// TwinCAT 3 PLC project Untitled1
// ProgramVersion: 3.1.4024.0
// CompilerDefines: VISU_USEWSTRING
// libraries:
//   CmpBitmapPool, * (System)
//   GearMotionBaseApplication, * (Beckhoff_sh Yuyang)
//   Tc2_EtherCAT, * (Beckhoff Automation GmbH)
//   Tc2_Math, * (Beckhoff Automation GmbH)
//   Tc2_MC2, * (Beckhoff Automation GmbH)
//   Tc2_MC2_Camming, * (Beckhoff Automation GmbH)
//   Tc2_Standard, * (Beckhoff Automation GmbH)
//   Tc2_System, * (Beckhoff Automation GmbH)
//   Tc2_Utilities, * (Beckhoff Automation GmbH)
//   Tc3_MC2_AdvancedHoming, * (Beckhoff Automation GmbH)
//   Tc3_Module, * (Beckhoff Automation GmbH)
//   VisuSymbols,3.5.10.0,System
// project tree:
//   / GlobalTextList.TcGTLO, PhysicalDisplay.TcIPO, VISU_TASK.TcTTO, Param.TcGVL, PlcTask.TcTTO, 视图管理器.TcVMO
//   Visus/ FB_Visus.TcPOU, Visualization.TcVIS
//   _04_Application/ MAIN.TcPOU
//   _03_MotionSystem/ FB_ShowMotion.TcPOU, I_ShowMotion.TcIO
// real-time tasks:
//   TASK PlcTask: cycle T#10ms, priority 20, ADS port 350
//   TASK VISU_TASK: cycle T#200000us, priority 30, ADS port 351
// motion (NC):
//   TASK NC-Task 1 SAF: cycle T#2ms, priority 4, ADS port 501
//   TASK NC-Task 1 SVB: cycle T#10ms, priority 8, ADS port 511
//   AXIS Axis 1_S (id 1)
//     Dynamic: Acceleration=14565, Deceleration=14565, Jerk=7282.5
//     Velo: RefSearch=291.3, RefSync=291.3, SlowManual=300, Fast=29130, Maximum=29130
//     OtherSettings: AllowMotionCmdToSlave=true
//     encoder EncType=1
//       EncPara: ScaleFactorNumerator=360, ScaleFactorDenominator=1048576, Offset=4873.63
//     drive DrvType=5
//       Analog: VeloReferenz=32043, TorqueSetpointScale=10, ScaleFactorActTorque=0.1
//       TimeComp: TaskDelayCycles=1
//     controller CtrType=1
//       CtrPara: PriorControlFactor=1
//         Observer: BandWidth=20
//   AXIS Axis 2_E (id 2)
//     Dynamic: Acceleration=14565, Deceleration=14565, Jerk=7282.5
//     Velo: RefSearch=291.3, RefSync=291.3, SlowManual=300, Fast=29130, Maximum=29130
//     OtherSettings: AllowMotionCmdToSlave=true
//     encoder EncType=1
//       EncPara: ScaleFactorNumerator=360, ScaleFactorDenominator=1048576, Offset=-6850.4
//     drive DrvType=5
//       Analog: VeloReferenz=32043, TorqueSetpointScale=10, ScaleFactorActTorque=0.1
//       TimeComp: TaskDelayCycles=1
//     controller CtrType=1
//       CtrPara: PriorControlFactor=1
//         Observer: BandWidth=20
//   AXIS Axis 3_R (id 3)
//     Dynamic: Acceleration=43695, Deceleration=43695, Jerk=131085
//     Velo: RefSearch=291.3, RefSync=291.3, SlowManual=1456.5, FastManual=8739, Fast=29130, Maximum=29130
//     OtherSettings: AllowMotionCmdToSlave=true
//     encoder EncType=1
//       EncPara: ScaleFactorNumerator=360, ScaleFactorDenominator=1048576, Offset=-4097.87
//     drive DrvType=5
//       Analog: VeloReferenz=32043, TorqueSetpointScale=10, ScaleFactorActTorque=0.1
//       TimeComp: TaskDelayCycles=1
//     controller CtrType=1
//       CtrPara: PriorControlFactor=1
//         PosDiffControl: Enable=false
//         Observer: BandWidth=20
//   AXIS Axis 4_V (id 4)
//     Dynamic: Acceleration=14565, Deceleration=14565, Jerk=7282.5
//     Velo: RefSearch=291.3, RefSync=291.3, SlowManual=300, Fast=29130, Maximum=29130
//     OtherSettings: AllowMotionCmdToSlave=true
//     encoder EncType=1
//       EncPara: ScaleFactorNumerator=360, ScaleFactorDenominator=1048576, Offset=-3588.52
//     drive DrvType=5
//       Analog: VeloReferenz=32043, TorqueSetpointScale=10, ScaleFactorActTorque=0.1
//       TimeComp: TaskDelayCycles=1
//     controller CtrType=1
//       CtrPara: PriorControlFactor=1
//         Observer: BandWidth=20
//   AXIS Axis 5_O (id 5)
//     Dynamic: Acceleration=14565, Deceleration=14565, Jerk=7282.5
//     Velo: RefSearch=291.3, RefSync=291.3, SlowManual=300, Fast=29130, Maximum=29130
//     OtherSettings: AllowMotionCmdToSlave=true
//     encoder EncType=1
//       EncPara: ScaleFactorNumerator=360, ScaleFactorDenominator=1048576, Offset=-612.17
//     drive DrvType=5
//       Analog: VeloReferenz=32043, TorqueSetpointScale=10, ScaleFactorActTorque=0.1
//       TimeComp: TaskDelayCycles=1
//     controller CtrType=1
//       CtrPara: PriorControlFactor=1
//         Observer: BandWidth=20
//   AXIS Axis 6 (id 6)
//     OtherSettings: AllowMotionCmdToSlave=true
//     encoder EncType=19
//       EncPara: MaxCount=#xffffffff
//     drive DrvType=16
//       DrvPara: MaxCount=#xffffffff, DriveControlDWord=#x00000100
//         Analog: TorqueSetpointScale=10, ScaleFactorActTorque=0.1
//         TimeComp: TaskDelayCycles=1
//     controller CtrType=1
//       CtrPara: PriorControlFactor=1
//         Observer: BandWidth=20
//   AXIS Axis 7 (id 7)
//     OtherSettings: AllowMotionCmdToSlave=true
//     encoder EncType=19
//       EncPara: MaxCount=#xffffffff
//     drive DrvType=16
//       DrvPara: MaxCount=#xffffffff, DriveControlDWord=#x00000100
//         Analog: TorqueSetpointScale=10, ScaleFactorActTorque=0.1
//         TimeComp: TaskDelayCycles=1
//     controller CtrType=1
//       CtrPara: PriorControlFactor=1
//         Observer: BandWidth=20
//   AXIS Axis 8 (id 8)
//     OtherSettings: AllowMotionCmdToSlave=true
//     encoder EncType=19
//       EncPara: MaxCount=#xffffffff
//     drive DrvType=16
//       DrvPara: MaxCount=#xffffffff, DriveControlDWord=#x00000100
//         Analog: TorqueSetpointScale=10, ScaleFactorActTorque=0.1
//         TimeComp: TaskDelayCycles=1
//     controller CtrType=1
//       CtrPara: PriorControlFactor=1
//         Observer: BandWidth=20
// variable links:
//   Untitled1/Untitled1 Instance <-> NC-Task 1 SAF/Axes/Axis 1_S
//     PlcTask Inputs/MAIN.fbShowMotion.Axisinstance[1].NcToPlc <-> Outputs/ToPlc
//     PlcTask Inputs/MAIN.fbVisus.ArrAxisNotMoving[1] <-> Outputs/ToPlc/StateDWord/NotMoving
//     PlcTask Inputs/MAIN.fbVisus.ArrAxisPosition[1] <-> Outputs/ToPlc/ActPos
//     PlcTask Outputs/MAIN.fbShowMotion.Axisinstance[1].PlcToNc <-> Inputs/FromPlc
//   Untitled1/Untitled1 Instance <-> NC-Task 1 SAF/Axes/Axis 2_E
//     PlcTask Inputs/MAIN.fbShowMotion.Axisinstance[2].NcToPlc <-> Outputs/ToPlc
//     PlcTask Inputs/MAIN.fbVisus.ArrAxisNotMoving[2] <-> Outputs/ToPlc/StateDWord/NotMoving
//     PlcTask Inputs/MAIN.fbVisus.ArrAxisPosition[2] <-> Outputs/ToPlc/ActPos
//     PlcTask Outputs/MAIN.fbShowMotion.Axisinstance[2].PlcToNc <-> Inputs/FromPlc
//   Untitled1/Untitled1 Instance <-> NC-Task 1 SAF/Axes/Axis 3_R
//     PlcTask Inputs/MAIN.fbShowMotion.Axisinstance[3].NcToPlc <-> Outputs/ToPlc
//     PlcTask Inputs/MAIN.fbVisus.ArrAxisNotMoving[3] <-> Outputs/ToPlc/StateDWord/NotMoving
//     PlcTask Inputs/MAIN.fbVisus.ArrAxisPosition[3] <-> Outputs/ToPlc/ActPos
//     PlcTask Outputs/MAIN.fbShowMotion.Axisinstance[3].PlcToNc <-> Inputs/FromPlc
//   Untitled1/Untitled1 Instance <-> NC-Task 1 SAF/Axes/Axis 4_V
//     PlcTask Inputs/MAIN.fbShowMotion.Axisinstance[4].NcToPlc <-> Outputs/ToPlc
//     PlcTask Inputs/MAIN.fbVisus.ArrAxisNotMoving[4] <-> Outputs/ToPlc/StateDWord/NotMoving
//     PlcTask Inputs/MAIN.fbVisus.ArrAxisPosition[4] <-> Outputs/ToPlc/ActPos
//     PlcTask Outputs/MAIN.fbShowMotion.Axisinstance[4].PlcToNc <-> Inputs/FromPlc
//   Untitled1/Untitled1 Instance <-> NC-Task 1 SAF/Axes/Axis 5_O
//     PlcTask Inputs/MAIN.fbShowMotion.Axisinstance[5].NcToPlc <-> Outputs/ToPlc
//     PlcTask Inputs/MAIN.fbVisus.ArrAxisNotMoving[5] <-> Outputs/ToPlc/StateDWord/NotMoving
//     PlcTask Inputs/MAIN.fbVisus.ArrAxisPosition[5] <-> Outputs/ToPlc/ActPos
//     PlcTask Outputs/MAIN.fbShowMotion.Axisinstance[5].PlcToNc <-> Inputs/FromPlc

CONFIGURATION Untitled1
    RESOURCE PLC ON TwinCAT3
        TASK VISU_TASK(INTERVAL := T#200000us, PRIORITY := 30);
        TASK PlcTask(INTERVAL := T#10ms, PRIORITY := 20);
        PROGRAM VisuElems_Visu_Prg WITH VISU_TASK : VisuElems.Visu_Prg;
        PROGRAM MAIN WITH PlcTask : MAIN;
    END_RESOURCE
END_CONFIGURATION

// ---- Param.TcGVL
{attribute 'qualified_only'}
VAR_GLOBAL CONSTANT
	CamTablePoints											: INT		:= 10;		// 凸轮表点位个数 
	MIN_SLAVES												: 	UINT  := 1;
	MAX_SLAVES												: 	UINT  := 1000;
	MIN_ANALOGVALUE											:	LREAL := 0;
	MAX_ANALOGVALUE											:	LREAL := 32767;
	TimeZone                 							    :   INT   := 30;			// FB_SignalAlarmRecord
	MaxReadSizeBuff											: UDINT		:= 1024;
END_VAR

// ---- _03_MotionSystem/I_ShowMotion.TcIO
// Demo接口
INTERFACE I_ShowMotion EXTENDS I_Base

PROPERTY P_Reset : BOOL
GET
END_GET
SET
END_SET
END_PROPERTY

// 如果为TRUE，启动运行
PROPERTY P_Start : BOOL
GET
END_GET
SET
END_SET
END_PROPERTY

// 如果为TRUE，则停止运动
PROPERTY P_Stop : BOOL
GET
END_GET
SET
END_SET
END_PROPERTY

// 运动模式
PROPERTY ShowPattern : INT
GET
END_GET
SET
END_SET
END_PROPERTY

END_INTERFACE

// ---- _04_Application/MAIN.TcPOU
PROGRAM MAIN
VAR
	fbVisus						: FB_Visus;
	
	bStart						: BOOL		:=TRUE;
	bStop						: BOOL;
	bReset						: BOOL;
	
	// 对象实例
	fbShowMotion				: FB_ShowMotion;	
	
	// 接口
	iShowMotion					: I_ShowMotion			:= fbShowMotion;
	iShowRuntime				: I_Runtime				:= fbShowMotion;
	iVisusRuntime				: I_Runtime				:= fbVisus;
END_VAR

iShowRuntime.Cyclic();

// 设置运动方式

iShowMotion.ShowPattern	:= 2;

// 启动
IF bStart THEN
	iShowMotion.P_Start	:= TRUE;
	bStart:= FALSE;
END_IF
IF bStop THEN
	iShowMotion.P_Stop	:= TRUE;
	 bStop:= FALSE;
END_IF
IF bReset THEN
	iShowMotion.P_Reset	:= TRUE;
	bReset	:= FALSE;
END_IF

// HMI
iVisusRuntime.Cyclic();

END_PROGRAM

// ---- Visus/FB_Visus.TcPOU
FUNCTION_BLOCK FB_Visus IMPLEMENTS  I_Runtime

VAR
	ArrAxisPosition				AT%I* : ARRAY [1..5] OF LREAL;
	ArrAxisNotMoving			AT%I* : ARRAY [1..5] OF BOOL;	
END_VAR

METHOD Cyclic
//
END_METHOD

END_FUNCTION_BLOCK

// ---- _03_MotionSystem/FB_ShowMotion.TcPOU
// Demo对象
FUNCTION_BLOCK FB_ShowMotion IMPLEMENTS I_ShowMotion, I_Runtime

VAR
	_ShowPattern		: INT;													// 运动模式

	Axisinstance		: ARRAY [1..5] OF FB_GearNcAxis;						// 带有特殊齿轮相位回原工艺的轴类型实例

	iAxis				: ARRAY [1..5] OF  I_Axis;								// 基本轴接口
	iGearHome			: ARRAY [1..5] OF I_GearHome;							// 相位回原接口
		
	iCamTableAxis2		: I_CamTable;											// 从轴2的凸轮表接口
	iCamTableAxis3		: I_CamTable;											// 从轴3的凸轮表接口
	iCamTableAxis4		: I_CamTable;											// 从轴4的凸轮表接口
	
	CamTableAxis2		: FB_CamTable;											// 从轴2的凸轮表实例
	CamTableAxis3		: FB_CamTable;											// 从轴3的凸轮表实例
	CamTableAxis4		: FB_CamTable;											// 从轴4的凸轮表实例
	
	TargetVelFast		: ST_axis_Vel				:=(Axis_Vel := 200, Axis_Acc := 6000, Axis_Dec := 6000, Axis_Jerk := 40000);	// 快速参数
	TargetVelSlow		: ST_axis_Vel				:=(Axis_Vel := 100, Axis_Acc := 6000, Axis_Dec := 6000, Axis_Jerk := 40000);	// 慢速参数

	statecase			: INT := 999;	
	Resetstatecase		: INT := 10;											
	Homestatecase		: INT := 10;
	
	delayton			: TON;													// 延时功能块
	movingMonitor		: TON;													// 监控未移动时间的功能块
	HomingMonitor		: TON;													// 监控回原时间的功能块
	
	bStop				: BOOL;													// 如果为TRUE，则停止运动										
	bReset				: BOOL;													// 如果为TRUE，复位
	bStart				: BOOL;													// 如果为TRUE，启动运行

	bCamSwitch			: BOOL;													// 如果为TRUE，则允许耦合凸轮表
	binited				: BOOL;													// 如果为TRUE，则已经初始化完成，创建完凸轮表
	Error				: BOOL;													// 如果为TRUE，则有轴组产生错误
	bHomeDone			: BOOL;													// 如果为TRUE，则回原完成
END_VAR

// 回原
METHOD PROTECTED AxisesHome : BOOL
VAR_INPUT
END_VAR
VAR
	index		: INT;
	Queryindex		: INT;
	DistanceAxis1TogoBw: LREAL;
	DistanceAxis1TogoFw: LREAL;
END_VAR

VAR_INST
END_VAR
CASE Homestatecase OF 
	
10:
// 回原过程中保持使能
FOR index	:= 1 TO 5 DO
	iAxis[index].Power(TRUE);
END_FOR

Homestatecase	:= 11;

11:
// 判断轴组是否实现了相位回原的接口，如果实现进行转换，跳到12步进行特殊相位回原
FOR Queryindex	:= 1 TO 5 DO
	IF __QUERYINTERFACE(iAxis[Queryindex],iGearHome[Queryindex]) THEN 

		Homestatecase	:= 12;
	
	ELSE
		RETURN;
	END_IF
END_FOR

// 360/8=45； 对轴1进行最近符合相位的回原
12:
IF  iGearHome[1].GearHome(45) THEN
	Homestatecase	:= 13;
END_IF

// 对轴5进行最近符合相位的回原
13:
IF iGearHome[5].GearHome(45) THEN
	Homestatecase	:= 14;
END_IF

// 对轴2进行最近符合相位的回原
14:
IF iGearHome[2].GearHome(45) THEN
	Homestatecase	:= 15;
END_IF

// 对轴4进行最近符合相位的回原
15:
IF iGearHome[4].GearHome(45) THEN
	Homestatecase	:= 16;
END_IF

// 对轴3进行最近符合相位的回原
16:
IF iGearHome[3].GearHome(45) THEN
	Homestatecase	:= 19;
END_IF

// 相位在可以耦合的位置之后，先将其他轴耦合轴2
19:
iAxis[1].GearIn(TRUE, iAxis[2],-1,1);
iAxis[3].GearIn(TRUE, iAxis[2],-1,1);
iAxis[4].GearIn(TRUE, iAxis[2], 1,1);
iAxis[5].GearIn(TRUE, iAxis[2],-1,1);


delayton(IN:=TRUE,PT:=T#1S);
IF delayton.Q THEN
	delayton(IN:=FALSE,PT:=T#1S);
	Homestatecase	:= 20;
END_IF

// 单独对轴2进行回原
20:
iAxis[1].GearIn(FALSE, iAxis[2],-1,1);
iAxis[3].GearIn(FALSE, iAxis[2],-1,1);
iAxis[4].GearIn(FALSE, iAxis[2], 1,1);
iAxis[5].GearIn(FALSE, iAxis[2],-1,1);

IF iAxis[2].MoveAbs(TRUE,0,TargetVelSlow) THEN
	iAxis[2].MoveAbs(FALSE,0,TargetVelSlow);
	Homestatecase	:= 30;
END_IF

// 轴2回原之后，解耦
30:
IF iAxis[1].GearOut(TRUE) THEN
	IF iAxis[3].GearOut(TRUE) THEN
		IF iAxis[4].GearOut(TRUE) THEN
			IF iAxis[5].GearOut(TRUE) THEN
				iAxis[1].GearOut(FALSE);
				iAxis[3].GearOut(FALSE);
				iAxis[4].GearOut(FALSE);
				iAxis[5].GearOut(FALSE);
				Homestatecase	:= 40;
			END_IF
		END_IF
	END_IF
END_IF

// 单独对轴1进行回原
40:
IF iAxis[1].MoveAbs(TRUE,0,TargetVelSlow) THEN
	iAxis[1].MoveAbs(FALSE,0,TargetVelSlow);
	Homestatecase	:= 60;
END_IF

// 将轴4相邻的轴3和5对轴4进行耦合
60:
iAxis[3].GearIn(TRUE, iAxis[4],-1,1);
iAxis[5].GearIn(TRUE, iAxis[4],-1,1);

// 单独对轴4进行回原
IF iAxis[4].MoveAbs(TRUE,0,TargetVelSlow) THEN
	iAxis[4].MoveAbs(FALSE,0,TargetVelSlow);
	iAxis[3].GearIn(FALSE, iAxis[4],-1,1);
	iAxis[5].GearIn(FALSE, iAxis[4],-1,1);
	Homestatecase	:= 70;
END_IF

// 轴4回原之后解耦35
70:
IF iAxis[3].GearOut(TRUE) THEN
	IF iAxis[5].GearOut(TRUE) THEN
		iAxis[3].GearOut(FALSE);
		iAxis[5].GearOut(FALSE);		
		Homestatecase	:= 80;
	END_IF
END_IF

// 分别对轴35进行回原
80:
IF iAxis[3].MoveAbs(TRUE,0,TargetVelSlow) AND 
	iAxis[5].MoveAbs(TRUE,0,TargetVelSlow) THEN
	iAxis[3].MoveAbs(FALSE,0,TargetVelSlow);
	iAxis[5].MoveAbs(FALSE,0,TargetVelSlow);
	bHomeDone	:= AxisesHome:= TRUE;
	Homestatecase	:= 10;
END_IF

END_CASE
END_METHOD

METHOD Cyclic

VAR
	index: INT;
END_VAR
// 检查轴状态
FOR index	:= 1 TO 5 DO
	iAxis[index].CyclicCheck();
END_FOR

// 传递报错
Error	:= iAxis[1].AxesStatus.Error OR iAxis[2].AxesStatus.Error OR iAxis[3].AxesStatus.Error 	OR
		   iAxis[4].AxesStatus.Error OR iAxis[5].AxesStatus.Error;

// 根据	_ShowPattern 的值选择运动的方式	   
IF _ShowPattern = 1 THEN
	MotionPattern1();
ELSIF _ShowPattern = 2 THEN 
	MotionPattern2();
ELSIF _ShowPattern = 3 THEN
	MotionPattern3();
END_IF
END_METHOD

METHOD PROTECTED EditCamPoints
VAR_INPUT
END_VAR
// 凸轮表1:轴2点位
iCamTableAxis2.rCamData[1].PointIndex 			:= 1 ;
iCamTableAxis2.rCamData[1].FunctionType			:= MOTIONFUNCTYPE_POLYNOM1;
iCamTableAxis2.rCamData[1].PointType			:= MOTIONPOINTTYPE_MOTION;
iCamTableAxis2.rCamData[1].RelIndexNextPoint	:= 1;     
iCamTableAxis2.rCamData[1].MasterPos			:= 0;
iCamTableAxis2.rCamData[1].SlavePos				:= 0;
iCamTableAxis2.rCamData[1].SlaveVelo			:= 1;
iCamTableAxis2.rCamData[1].SlaveAcc				:= 0;
iCamTableAxis2.rCamData[1].SlaveJerk			:= 0;

iCamTableAxis2.rCamData[2].PointIndex 			:= 2 ;
iCamTableAxis2.rCamData[2].FunctionType			:= MOTIONFUNCTYPE_POLYNOM1;
iCamTableAxis2.rCamData[2].PointType			:= MOTIONPOINTTYPE_MOTION;
iCamTableAxis2.rCamData[2].RelIndexNextPoint	:= 1;    	
iCamTableAxis2.rCamData[2].MasterPos			:= 360;
iCamTableAxis2.rCamData[2].SlavePos				:= 0;
iCamTableAxis2.rCamData[2].SlaveVelo			:= 1;
iCamTableAxis2.rCamData[2].SlaveAcc				:= 0;
iCamTableAxis2.rCamData[2].SlaveJerk			:= 0;

iCamTableAxis2.rCamData[3].PointIndex 			:= 3;
iCamTableAxis2.rCamData[3].FunctionType			:= MOTIONFUNCTYPE_POLYNOM1;
iCamTableAxis2.rCamData[3].PointType			:= MOTIONPOINTTYPE_MOTION;
iCamTableAxis2.rCamData[3].RelIndexNextPoint	:= 1;    	
iCamTableAxis2.rCamData[3].MasterPos			:= 1440;
iCamTableAxis2.rCamData[3].SlavePos				:= -1080;
iCamTableAxis2.rCamData[3].SlaveVelo			:= 1;
iCamTableAxis2.rCamData[3].SlaveAcc				:= 0;
iCamTableAxis2.rCamData[3].SlaveJerk			:= 0;

iCamTableAxis2.rCamData[4].PointIndex 			:= 4;
iCamTableAxis2.rCamData[4].FunctionType			:= MOTIONFUNCTYPE_POLYNOM1;
iCamTableAxis2.rCamData[4].PointType			:= MOTIONPOINTTYPE_MOTION;
iCamTableAxis2.rCamData[4].RelIndexNextPoint	:= 1;    	
iCamTableAxis2.rCamData[4].MasterPos			:= 2160;
iCamTableAxis2.rCamData[4].SlavePos				:= -1080;
iCamTableAxis2.rCamData[4].SlaveVelo			:= 1;
iCamTableAxis2.rCamData[4].SlaveAcc				:= 0;
iCamTableAxis2.rCamData[4].SlaveJerk			:= 0;

iCamTableAxis2.rCamData[5].PointIndex 			:= 5;
iCamTableAxis2.rCamData[5].FunctionType			:= MOTIONFUNCTYPE_POLYNOM1;
iCamTableAxis2.rCamData[5].PointType			:= MOTIONPOINTTYPE_MOTION;
iCamTableAxis2.rCamData[5].RelIndexNextPoint	:= 1;    	
iCamTableAxis2.rCamData[5].MasterPos			:= 2340;
iCamTableAxis2.rCamData[5].SlavePos				:= -1260;
iCamTableAxis2.rCamData[5].SlaveVelo			:= 1;
iCamTableAxis2.rCamData[5].SlaveAcc				:= 0;
iCamTableAxis2.rCamData[5].SlaveJerk			:= 0;

iCamTableAxis2.rCamData[6].PointIndex 			:= 6;
iCamTableAxis2.rCamData[6].FunctionType			:= MOTIONFUNCTYPE_POLYNOM1;
iCamTableAxis2.rCamData[6].PointType			:= MOTIONPOINTTYPE_MOTION;
iCamTableAxis2.rCamData[6].RelIndexNextPoint	:= 1;    	
iCamTableAxis2.rCamData[6].MasterPos			:= 3060;
iCamTableAxis2.rCamData[6].SlavePos				:= -1260;
iCamTableAxis2.rCamData[6].SlaveVelo			:= 1;
iCamTableAxis2.rCamData[6].SlaveAcc				:= 0;
iCamTableAxis2.rCamData[6].SlaveJerk			:= 0;

iCamTableAxis2.rCamData[7].PointIndex 			:= 7;
iCamTableAxis2.rCamData[7].FunctionType			:= MOTIONFUNCTYPE_POLYNOM1;
iCamTableAxis2.rCamData[7].PointType			:= MOTIONPOINTTYPE_MOTION;
iCamTableAxis2.rCamData[7].RelIndexNextPoint	:= 1;    	
iCamTableAxis2.rCamData[7].MasterPos			:= 3240;
iCamTableAxis2.rCamData[7].SlavePos				:= -1440;
iCamTableAxis2.rCamData[7].SlaveVelo			:= 1;
iCamTableAxis2.rCamData[7].SlaveAcc				:= 0;
iCamTableAxis2.rCamData[7].SlaveJerk			:= 0;

iCamTableAxis2.rCamData[8].PointIndex 			:= 8;
iCamTableAxis2.rCamData[8].FunctionType			:= MOTIONFUNCTYPE_POLYNOM1;
iCamTableAxis2.rCamData[8].PointType			:= MOTIONPOINTTYPE_MOTION;
iCamTableAxis2.rCamData[8].RelIndexNextPoint	:= 1;    	
iCamTableAxis2.rCamData[8].MasterPos			:= 3960;
iCamTableAxis2.rCamData[8].SlavePos				:= -1440;
iCamTableAxis2.rCamData[8].SlaveVelo			:= 1;
iCamTableAxis2.rCamData[8].SlaveAcc				:= 0;
iCamTableAxis2.rCamData[8].SlaveJerk			:= 0;

iCamTableAxis2.rCamData[9].PointIndex 			:= 9;
iCamTableAxis2.rCamData[9].FunctionType			:= MOTIONFUNCTYPE_POLYNOM1;
iCamTableAxis2.rCamData[9].PointType			:= MOTIONPOINTTYPE_MOTION;
iCamTableAxis2.rCamData[9].RelIndexNextPoint	:= 1;    	
iCamTableAxis2.rCamData[9].MasterPos			:= 4320;
iCamTableAxis2.rCamData[9].SlavePos				:= -1800;
iCamTableAxis2.rCamData[9].SlaveVelo			:= 1;
iCamTableAxis2.rCamData[9].SlaveAcc				:= 0;
iCamTableAxis2.rCamData[9].SlaveJerk			:= 0;

iCamTableAxis2.rCamData[10].PointIndex 			:= 10;
iCamTableAxis2.rCamData[10].FunctionType		:= MOTIONFUNCTYPE_POLYNOM1;
iCamTableAxis2.rCamData[10].PointType			:= MOTIONPOINTTYPE_MOTION;
iCamTableAxis2.rCamData[10].RelIndexNextPoint	:= 0;    	
iCamTableAxis2.rCamData[10].MasterPos			:= 5040;
iCamTableAxis2.rCamData[10].SlavePos			:= -1800;
iCamTableAxis2.rCamData[10].SlaveVelo			:= 1;
iCamTableAxis2.rCamData[10].SlaveAcc			:= 0;
iCamTableAxis2.rCamData[10].SlaveJerk			:= 0;






// 凸轮表2：轴3点位
iCamTableAxis3.rCamData[1].PointIndex 			:= 1 ;
iCamTableAxis3.rCamData[1].FunctionType			:= MOTIONFUNCTYPE_POLYNOM1;
iCamTableAxis3.rCamData[1].PointType			:= MOTIONPOINTTYPE_MOTION;
iCamTableAxis3.rCamData[1].RelIndexNextPoint	:= 1;     
iCamTableAxis3.rCamData[1].MasterPos			:= 0;
iCamTableAxis3.rCamData[1].SlavePos				:= 0;
iCamTableAxis3.rCamData[1].SlaveVelo			:= 1;
iCamTableAxis3.rCamData[1].SlaveAcc				:= 0;
iCamTableAxis3.rCamData[1].SlaveJerk			:= 0;

iCamTableAxis3.rCamData[2].PointIndex 			:= 2 ;
iCamTableAxis3.rCamData[2].FunctionType			:= MOTIONFUNCTYPE_POLYNOM1;
iCamTableAxis3.rCamData[2].PointType			:= MOTIONPOINTTYPE_MOTION;
iCamTableAxis3.rCamData[2].RelIndexNextPoint	:= 1;    	
iCamTableAxis3.rCamData[2].MasterPos			:= 360;
iCamTableAxis3.rCamData[2].SlavePos				:= 0;
iCamTableAxis3.rCamData[2].SlaveVelo			:= 1;
iCamTableAxis3.rCamData[2].SlaveAcc				:= 0;
iCamTableAxis3.rCamData[2].SlaveJerk			:= 0;

iCamTableAxis3.rCamData[3].PointIndex 			:= 3;
iCamTableAxis3.rCamData[3].FunctionType			:= MOTIONFUNCTYPE_POLYNOM1;
iCamTableAxis3.rCamData[3].PointType			:= MOTIONPOINTTYPE_MOTION;
iCamTableAxis3.rCamData[3].RelIndexNextPoint	:= 0;    	
iCamTableAxis3.rCamData[3].MasterPos			:= 1440;
iCamTableAxis3.rCamData[3].SlavePos				:= 1080;
iCamTableAxis3.rCamData[3].SlaveVelo			:= 1;
iCamTableAxis3.rCamData[3].SlaveAcc				:= 0;
iCamTableAxis3.rCamData[3].SlaveJerk			:= 0;

iCamTableAxis3.rCamData[4].PointIndex 			:= 4;
iCamTableAxis3.rCamData[4].FunctionType			:= MOTIONFUNCTYPE_POLYNOM1;
iCamTableAxis3.rCamData[4].PointType			:= MOTIONPOINTTYPE_MOTION;
iCamTableAxis3.rCamData[4].RelIndexNextPoint	:= 1;    	
iCamTableAxis3.rCamData[4].MasterPos			:= 2160;
iCamTableAxis3.rCamData[4].SlavePos				:= 1080;
iCamTableAxis3.rCamData[4].SlaveVelo			:= 1;
iCamTableAxis3.rCamData[4].SlaveAcc				:= 0;
iCamTableAxis3.rCamData[4].SlaveJerk			:= 0;

iCamTableAxis3.rCamData[5].PointIndex 			:= 5;
iCamTableAxis3.rCamData[5].FunctionType			:= MOTIONFUNCTYPE_POLYNOM1;
iCamTableAxis3.rCamData[5].PointType			:= MOTIONPOINTTYPE_MOTION;
iCamTableAxis3.rCamData[5].RelIndexNextPoint	:= 1;    	
iCamTableAxis3.rCamData[5].MasterPos			:= 2340;
iCamTableAxis3.rCamData[5].SlavePos				:= 1260;
iCamTableAxis3.rCamData[5].SlaveVelo			:= 1;
iCamTableAxis3.rCamData[5].SlaveAcc				:= 0;
iCamTableAxis3.rCamData[5].SlaveJerk			:= 0;

iCamTableAxis3.rCamData[6].PointIndex 			:= 6;
iCamTableAxis3.rCamData[6].FunctionType			:= MOTIONFUNCTYPE_POLYNOM1;
iCamTableAxis3.rCamData[6].PointType			:= MOTIONPOINTTYPE_MOTION;
iCamTableAxis3.rCamData[6].RelIndexNextPoint	:= 1;    	
iCamTableAxis3.rCamData[6].MasterPos			:= 3060;
iCamTableAxis3.rCamData[6].SlavePos				:= 1260;
iCamTableAxis3.rCamData[6].SlaveVelo			:= 1;
iCamTableAxis3.rCamData[6].SlaveAcc				:= 0;
iCamTableAxis3.rCamData[6].SlaveJerk			:= 0;

iCamTableAxis3.rCamData[7].PointIndex 			:= 7;
iCamTableAxis3.rCamData[7].FunctionType			:= MOTIONFUNCTYPE_POLYNOM1;
iCamTableAxis3.rCamData[7].PointType			:= MOTIONPOINTTYPE_MOTION;
iCamTableAxis3.rCamData[7].RelIndexNextPoint	:= 1;    	
iCamTableAxis3.rCamData[7].MasterPos			:= 3240;
iCamTableAxis3.rCamData[7].SlavePos				:= 1440;
iCamTableAxis3.rCamData[7].SlaveVelo			:= 1;
iCamTableAxis3.rCamData[7].SlaveAcc				:= 0;
iCamTableAxis3.rCamData[7].SlaveJerk			:= 0;

iCamTableAxis3.rCamData[8].PointIndex 			:= 8;
iCamTableAxis3.rCamData[8].FunctionType			:= MOTIONFUNCTYPE_POLYNOM1;
iCamTableAxis3.rCamData[8].PointType			:= MOTIONPOINTTYPE_MOTION;
iCamTableAxis3.rCamData[8].RelIndexNextPoint	:= 0;    	
iCamTableAxis3.rCamData[8].MasterPos			:= 3960;
iCamTableAxis3.rCamData[8].SlavePos				:= 1440;
iCamTableAxis3.rCamData[8].SlaveVelo			:= 1;
iCamTableAxis3.rCamData[8].SlaveAcc				:= 0;
iCamTableAxis3.rCamData[8].SlaveJerk			:= 0;

iCamTableAxis3.rCamData[9].PointIndex 			:= 9;
iCamTableAxis3.rCamData[9].FunctionType			:= MOTIONFUNCTYPE_POLYNOM1;
iCamTableAxis3.rCamData[9].PointType			:= MOTIONPOINTTYPE_MOTION;
iCamTableAxis3.rCamData[9].RelIndexNextPoint	:= 1;    	
iCamTableAxis3.rCamData[9].MasterPos			:= 4320;
iCamTableAxis3.rCamData[9].SlavePos				:= 1800;
iCamTableAxis3.rCamData[9].SlaveVelo			:= 1;
iCamTableAxis3.rCamData[9].SlaveAcc				:= 0;
iCamTableAxis3.rCamData[9].SlaveJerk			:= 0;

iCamTableAxis3.rCamData[10].PointIndex 			:= 10;
iCamTableAxis3.rCamData[10].FunctionType		:= MOTIONFUNCTYPE_POLYNOM1;
iCamTableAxis3.rCamData[10].PointType			:= MOTIONPOINTTYPE_MOTION;
iCamTableAxis3.rCamData[10].RelIndexNextPoint	:= 0;    	
iCamTableAxis3.rCamData[10].MasterPos			:= 5040;
iCamTableAxis3.rCamData[10].SlavePos			:= 1800;
iCamTableAxis3.rCamData[10].SlaveVelo			:= 1;
iCamTableAxis3.rCamData[10].SlaveAcc			:= 0;
iCamTableAxis3.rCamData[10].SlaveJerk			:= 0;






// 凸轮表3：轴4点位
iCamTableAxis4.rCamData[1].PointIndex 			:= 1 ;
iCamTableAxis4.rCamData[1].FunctionType			:= MOTIONFUNCTYPE_POLYNOM1;
iCamTableAxis4.rCamData[1].PointType			:= MOTIONPOINTTYPE_MOTION;
iCamTableAxis4.rCamData[1].RelIndexNextPoint	:= 1;     
iCamTableAxis4.rCamData[1].MasterPos			:= 0;
iCamTableAxis4.rCamData[1].SlavePos				:= 0;
iCamTableAxis4.rCamData[1].SlaveVelo			:= 1;
iCamTableAxis4.rCamData[1].SlaveAcc				:= 0;
iCamTableAxis4.rCamData[1].SlaveJerk			:= 0;

iCamTableAxis4.rCamData[2].PointIndex 			:= 2 ;
iCamTableAxis4.rCamData[2].FunctionType			:= MOTIONFUNCTYPE_POLYNOM1;
iCamTableAxis4.rCamData[2].PointType			:= MOTIONPOINTTYPE_MOTION;
iCamTableAxis4.rCamData[2].RelIndexNextPoint	:= 1;    	
iCamTableAxis4.rCamData[2].MasterPos			:= 360;
iCamTableAxis4.rCamData[2].SlavePos				:= 0;
iCamTableAxis4.rCamData[2].SlaveVelo			:= 1;
iCamTableAxis4.rCamData[2].SlaveAcc				:= 0;
iCamTableAxis4.rCamData[2].SlaveJerk			:= 0;

iCamTableAxis4.rCamData[3].PointIndex 			:= 3;
iCamTableAxis4.rCamData[3].FunctionType			:= MOTIONFUNCTYPE_POLYNOM1;
iCamTableAxis4.rCamData[3].PointType			:= MOTIONPOINTTYPE_MOTION;
iCamTableAxis4.rCamData[3].RelIndexNextPoint	:= 0;    	
iCamTableAxis4.rCamData[3].MasterPos			:= 1440;
iCamTableAxis4.rCamData[3].SlavePos				:= -1080;
iCamTableAxis4.rCamData[3].SlaveVelo			:= 1;
iCamTableAxis4.rCamData[3].SlaveAcc				:= 0;
iCamTableAxis4.rCamData[3].SlaveJerk			:= 0;


iCamTableAxis4.rCamData[4].PointIndex 			:= 4;
iCamTableAxis4.rCamData[4].FunctionType			:= MOTIONFUNCTYPE_POLYNOM1;
iCamTableAxis4.rCamData[4].PointType			:= MOTIONPOINTTYPE_MOTION;
iCamTableAxis4.rCamData[4].RelIndexNextPoint	:= 1;    	
iCamTableAxis4.rCamData[4].MasterPos			:= 2160;
iCamTableAxis4.rCamData[4].SlavePos				:= -1080;
iCamTableAxis4.rCamData[4].SlaveVelo			:= 1;
iCamTableAxis4.rCamData[4].SlaveAcc				:= 0;
iCamTableAxis4.rCamData[4].SlaveJerk			:= 0;

iCamTableAxis4.rCamData[5].PointIndex 			:= 5;
iCamTableAxis4.rCamData[5].FunctionType			:= MOTIONFUNCTYPE_POLYNOM1;
iCamTableAxis4.rCamData[5].PointType			:= MOTIONPOINTTYPE_MOTION;
iCamTableAxis4.rCamData[5].RelIndexNextPoint	:= 1;    	
iCamTableAxis4.rCamData[5].MasterPos			:= 2340;
iCamTableAxis4.rCamData[5].SlavePos				:= -1260;
iCamTableAxis4.rCamData[5].SlaveVelo			:= 1;
iCamTableAxis4.rCamData[5].SlaveAcc				:= 0;
iCamTableAxis4.rCamData[5].SlaveJerk			:= 0;

iCamTableAxis4.rCamData[6].PointIndex 			:= 6;
iCamTableAxis4.rCamData[6].FunctionType			:= MOTIONFUNCTYPE_POLYNOM1;
iCamTableAxis4.rCamData[6].PointType			:= MOTIONPOINTTYPE_MOTION;
iCamTableAxis4.rCamData[6].RelIndexNextPoint	:= 1;    	
iCamTableAxis4.rCamData[6].MasterPos			:= 3060;
iCamTableAxis4.rCamData[6].SlavePos				:= -1260;
iCamTableAxis4.rCamData[6].SlaveVelo			:= 1;
iCamTableAxis4.rCamData[6].SlaveAcc				:= 0;
iCamTableAxis4.rCamData[6].SlaveJerk			:= 0;

iCamTableAxis4.rCamData[7].PointIndex 			:= 7;
iCamTableAxis4.rCamData[7].FunctionType			:= MOTIONFUNCTYPE_POLYNOM1;
iCamTableAxis4.rCamData[7].PointType			:= MOTIONPOINTTYPE_MOTION;
iCamTableAxis4.rCamData[7].RelIndexNextPoint	:= 1;    	
iCamTableAxis4.rCamData[7].MasterPos			:= 3240;
iCamTableAxis4.rCamData[7].SlavePos				:= -1440;
iCamTableAxis4.rCamData[7].SlaveVelo			:= 1;
iCamTableAxis4.rCamData[7].SlaveAcc				:= 0;
iCamTableAxis4.rCamData[7].SlaveJerk			:= 0;

iCamTableAxis4.rCamData[8].PointIndex 			:= 8;
iCamTableAxis4.rCamData[8].FunctionType			:= MOTIONFUNCTYPE_POLYNOM1;
iCamTableAxis4.rCamData[8].PointType			:= MOTIONPOINTTYPE_MOTION;
iCamTableAxis4.rCamData[8].RelIndexNextPoint	:= 0;    	
iCamTableAxis4.rCamData[8].MasterPos			:= 3960;
iCamTableAxis4.rCamData[8].SlavePos				:= -1440;
iCamTableAxis4.rCamData[8].SlaveVelo			:= 1;
iCamTableAxis4.rCamData[8].SlaveAcc				:= 0;
iCamTableAxis4.rCamData[8].SlaveJerk			:= 0;

iCamTableAxis4.rCamData[9].PointIndex 			:= 9;
iCamTableAxis4.rCamData[9].FunctionType			:= MOTIONFUNCTYPE_POLYNOM1;
iCamTableAxis4.rCamData[9].PointType			:= MOTIONPOINTTYPE_MOTION;
iCamTableAxis4.rCamData[9].RelIndexNextPoint	:= 1;    	
iCamTableAxis4.rCamData[9].MasterPos			:= 4320;
iCamTableAxis4.rCamData[9].SlavePos				:= -1800;
iCamTableAxis4.rCamData[9].SlaveVelo			:= 1;
iCamTableAxis4.rCamData[9].SlaveAcc				:= 0;
iCamTableAxis4.rCamData[9].SlaveJerk			:= 0;

iCamTableAxis4.rCamData[10].PointIndex 			:= 10;
iCamTableAxis4.rCamData[10].FunctionType		:= MOTIONFUNCTYPE_POLYNOM1;
iCamTableAxis4.rCamData[10].PointType			:= MOTIONPOINTTYPE_MOTION;
iCamTableAxis4.rCamData[10].RelIndexNextPoint	:= 0;    	
iCamTableAxis4.rCamData[10].MasterPos			:= 5040;
iCamTableAxis4.rCamData[10].SlavePos			:= -1800;
iCamTableAxis4.rCamData[10].SlaveVelo			:= 1;
iCamTableAxis4.rCamData[10].SlaveAcc			:= 0;
iCamTableAxis4.rCamData[10].SlaveJerk			:= 0;
END_METHOD

METHOD PROTECTED EditCamTable
VAR_INPUT
END_VAR
// 编辑凸轮表1：从轴2
iCamTableAxis2.rTable.pArray		:= iCamTableAxis2.PCamData;
iCamTableAxis2.rTable.ArraySize		:= SIZEOF(iCamTableAxis2.PCamData^);
iCamTableAxis2.rTable.TableType		:= MC_TABLETYPE_MOTIONFUNCTION;
iCamTableAxis2.rTable.NoOfRows		:= 10;
iCamTableAxis2.rTable.NoOfColumns 	:= 1;

// 编辑凸轮表2：从轴3
iCamTableAxis3.rTable.pArray		:= iCamTableAxis3.PCamData;
iCamTableAxis3.rTable.ArraySize		:= SIZEOF(iCamTableAxis3.PCamData^);
iCamTableAxis3.rTable.TableType		:= MC_TABLETYPE_MOTIONFUNCTION;
iCamTableAxis3.rTable.NoOfRows		:= 10;
iCamTableAxis3.rTable.NoOfColumns 	:= 1;

// 编辑凸轮表3：从轴4
iCamTableAxis4.rTable.pArray		:= iCamTableAxis4.PCamData;
iCamTableAxis4.rTable.ArraySize		:= SIZEOF(iCamTableAxis4.PCamData^);
iCamTableAxis4.rTable.TableType		:= MC_TABLETYPE_MOTIONFUNCTION;
iCamTableAxis4.rTable.NoOfRows		:= 10;
iCamTableAxis4.rTable.NoOfColumns 	:= 1;
END_METHOD

METHOD FB_init : BOOL
VAR_INPUT
	bInitRetains : BOOL; // if TRUE, the retain variables are initialized (warm start / cold start)
	bInCopyCode : BOOL;  // if TRUE, the instance afterwards gets moved into the copy code (online change)
END_VAR
VAR
	index: INT;
END_VAR
// 将轴对象指向轴接口
FOR index	:= 1 TO 5 DO
	iAxis[index]	:= Axisinstance[index];
	
	IF iAxis[index] = 0 THEN
		RETURN;
	END_IF
	
END_FOR

// 将凸轮表对象指向凸轮表接口
iCamTableAxis2	:= CamTableAxis2;
iCamTableAxis3	:= CamTableAxis3;
iCamTableAxis4	:= CamTableAxis4;

IF (iCamTableAxis2 = 0) OR (iCamTableAxis3 = 0) OR (iCamTableAxis4 = 0) THEN
	RETURN;
END_IF
END_METHOD

// 初始化
METHOD PROTECTED InitCamTable : BOOL
VAR_INPUT
END_VAR
delayton(IN:=TRUE,PT:=T#1S);
IF delayton.Q THEN
	delayton(IN:=FALSE,PT:=T#5S);
	// 编辑点位
	EditCamPoints();	
	// 编辑凸轮表
	EditCamTable();		
	// 生成凸轮表123
	IF iCamTableAxis2.Generate(TRUE,1,TRUE,0) AND 
	   iCamTableAxis3.Generate(TRUE,2,TRUE,0) AND 
	   iCamTableAxis4.Generate(TRUE,3,TRUE,0) THEN
		binited	:= TRUE;
		InitCamTable	:= TRUE;				
	ELSE
		RETURN;
	END_IF
END_IF
END_METHOD

// 运动模式1
METHOD PROTECTED MotionPattern1
VAR_INPUT
END_VAR

VAR
	index		: INT;
	
	
END_VAR

CASE statecase OF 
	
0:
statecase:=10;


10:
// 使能
FOR index	:= 1 TO 5 DO
	iAxis[index].Power(TRUE);
END_FOR

delayton(IN:=TRUE,PT:=T#1S);
IF delayton.Q THEN
	delayton(IN:=FALSE,PT:=T#1S);
	statecase:=15;
END_IF

15: 
 IF iAxis[1].MoveAbs(TRUE,0,TargetVelFast) AND iAxis[2].MoveAbs(TRUE,0,TargetVelFast) AND iAxis[3].MoveAbs(TRUE,0,TargetVelFast) 

	AND iAxis[4].MoveAbs(TRUE,0,TargetVelFast) AND iAxis[5].MoveAbs(TRUE,0,TargetVelFast) THEN
	
	iAxis[1].MoveAbs(FALSE,0,TargetVelFast);
	iAxis[2].MoveAbs(FALSE,0,TargetVelFast);
	iAxis[3].MoveAbs(FALSE,0,TargetVelFast);
	iAxis[4].MoveAbs(FALSE,0,TargetVelFast);
	iAxis[5].MoveAbs(FALSE,0,TargetVelFast);
	
	statecase:=20;
	
END_IF


20:
IF iAxis[1].MoveAbs(TRUE,-360,TargetVelFast)  THEN
	iAxis[1].MoveAbs(FALSE,-300,TargetVelFast);
	statecase:=30;
END_IF

30:
IF iAxis[3].MoveAbs(TRUE,-360,TargetVelFast)  THEN
	iAxis[3].MoveAbs(FALSE,-300,TargetVelFast);
	statecase:=34;
END_IF


34:
IF iAxis[5].MoveAbs(TRUE,-360,TargetVelFast)  THEN
	iAxis[5].MoveAbs(FALSE,-300,TargetVelFast);
	statecase:=36;
END_IF

36:
IF iAxis[5].MoveAbs(TRUE,0,TargetVelFast)  THEN
	iAxis[5].MoveAbs(FALSE,0,TargetVelFast);
	statecase:=40;
END_IF


40:
IF iAxis[3].MoveAbs(TRUE,0,TargetVelFast)  THEN
	iAxis[3].MoveAbs(FALSE,0,TargetVelFast);
	statecase:=44;
END_IF


44:
IF iAxis[1].MoveAbs(TRUE,0,TargetVelFast)  THEN
	iAxis[1].MoveAbs(FALSE,0,TargetVelFast);
	statecase:=62;
END_IF


 
62:
iAxis[3].GearIn(TRUE,iAxis[1],1,1);


IF  iAxis[1].MoveAbs(TRUE,720,TargetVelFast)THEN
	iAxis[1].MoveAbs(FALSE,720,TargetVelFast);
	statecase:=63;
END_IF


63:
iAxis[3].GearIn(FALSE,iAxis[1],1,1);

IF  iAxis[1].MoveAbs(TRUE,0,TargetVelFast)THEN
	iAxis[1].MoveAbs(FALSE,0,TargetVelFast);
	IF iAxis[3].GearOut(TRUE) THEN
		iAxis[3].GearOut(FALSE);
		statecase:=64;
	END_IF
END_IF

64:

iAxis[3].GearIn(TRUE,iAxis[5],1,1);

IF  iAxis[5].MoveAbs(TRUE,-720,TargetVelFast)THEN
	iAxis[5].MoveAbs(FALSE,-720,TargetVelFast);
	statecase:=65;
END_IF

65:

iAxis[3].GearIn(FALSE,iAxis[5],1,1);

IF  iAxis[5].MoveAbs(TRUE,0,TargetVelFast)THEN
	iAxis[5].MoveAbs(FALSE,0,TargetVelFast);
	IF iAxis[3].GearOut(TRUE) THEN
		iAxis[3].GearOut(FALSE);
		statecase:=66;
	END_IF
END_IF


66:
iAxis[2].GearIn(TRUE,iAxis[1],-1,1);
iAxis[3].GearIn(TRUE,iAxis[1],1,1);
iAxis[4].GearIn(TRUE,iAxis[1],-1,1);
iAxis[5].GearIn(TRUE,iAxis[1],1,1);
statecase:=67;

67:
iAxis[2].GearIn(FALSE,iAxis[1],-1,1);
iAxis[3].GearIn(FALSE,iAxis[1],1,1);
iAxis[4].GearIn(FALSE,iAxis[1],-1,1);
iAxis[5].GearIn(FALSE,iAxis[1],1,1);
statecase:=68;


68:
IF iAxis[1].MoveAbs(TRUE,1440,TargetVelFast) THEN
	iAxis[1].MoveAbs(FALSE,1440,TargetVelFast) ;
	statecase:=70;
END_IF
 
70:
IF iAxis[1].MoveAbs(TRUE,0,TargetVelFast) THEN
	iAxis[1].MoveAbs(FALSE,0,TargetVelFast) ;
	statecase:=80;
END_IF


80:
IF iAxis[2].GearOut(TRUE) THEN
	IF iAxis[3].GearOut(TRUE) THEN
		IF iAxis[4].GearOut(TRUE) THEN
			IF iAxis[5].GearOut(TRUE) THEN
				iAxis[2].GearOut(FALSE);
				iAxis[3].GearOut(FALSE);
				iAxis[4].GearOut(FALSE);
				iAxis[5].GearOut(FALSE);
				statecase:=90;
			END_IF
		END_IF
	END_IF
END_IF




 90: 
 	IF iAxis[2].Halt(TRUE) AND iAxis[3].Halt(TRUE) AND iAxis[4].Halt(TRUE) THEN
		iAxis[2].Halt(FALSE);
		iAxis[3].Halt(FALSE);
		iAxis[4].Halt(FALSE);
		statecase:=10; 
	END_IF



840:

IF AxisesHome() THEN
	statecase:=10;
END_IF

1000:
IF iAxis[1].Stop(TRUE) AND iAxis[2].Stop(TRUE) AND iAxis[3].Stop(TRUE) AND iAxis[4].Stop(TRUE) AND iAxis[5].Stop(TRUE) THEN
	iAxis[1].Stop(FALSE);
	iAxis[2].Stop(FALSE);
	iAxis[3].Stop(FALSE);
	iAxis[4].Stop(FALSE);
	iAxis[5].Stop(FALSE);	
END_IF
	
1010:
IF iAxis[1].Reset(TRUE) AND iAxis[2].Reset(TRUE) AND iAxis[3].Reset(TRUE) AND iAxis[4].Reset(TRUE) AND iAxis[5].Reset(TRUE) THEN
	iAxis[1].Reset(FALSE);
	iAxis[2].Reset(FALSE);
	iAxis[3].Reset(FALSE);
	iAxis[4].Reset(FALSE);
	iAxis[5].Reset(FALSE);	
END_IF

END_CASE



IF bStop THEN
	statecase:=1000;
	bStop	:= FALSE;
END_IF

IF bReset THEN
	statecase:=1010;
	bReset	:= FALSE;
END_IF

IF bStart THEN
	statecase:=0;
	bStart	:= FALSE;
END_IF

movingMonitor(in:=iAxis[1].AxesStatus.NotMoving AND (statecase=20) ,PT:=T#5S);
IF movingMonitor.Q  THEN
	iAxis[1].MoveAbs(FALSE,0,TargetVelFast);
	iAxis[2].MoveAbs(FALSE,0,TargetVelFast);
	iAxis[3].MoveAbs(FALSE,0,TargetVelFast);
	iAxis[4].MoveAbs(FALSE,0,TargetVelFast);
	iAxis[5].MoveAbs(FALSE,0,TargetVelFast);
	statecase:=800;
END_IF

IF Error THEN
	delayton(IN:=TRUE,PT:=T#3S);
	IF delayton.Q THEN
		delayton(IN:=FALSE,PT:=T#3S);
		statecase:=800;
	END_IF
END_IF
END_METHOD

// 运动模式2
METHOD PROTECTED MotionPattern2
VAR_INPUT
END_VAR
VAR
	index: INT;
END_VAR

CASE statecase OF 

// 初始化	
0:
IF NOT binited THEN
	IF InitCamTable() THEN
		statecase:=10;
	END_IF	
ELSE
	statecase:=10;
END_IF

// 使能
10:
FOR index	:= 1 TO 5 DO
	iAxis[index].Power(TRUE);
END_FOR
delayton(IN:=TRUE,PT:=T#1S);
IF delayton.Q THEN
	delayton(IN:=FALSE,PT:=T#1S);
	statecase:=15;
END_IF

// 回原
15: 
 IF AxisesHome() THEN	
	statecase:=20;	
END_IF

// 将轴1运动到指定位置
20:
IF iAxis[1].MoveAbs(TRUE,-360,TargetVelFast)  THEN
	iAxis[1].MoveAbs(FALSE,-300,TargetVelFast);
	statecase:=30;
END_IF

// 将轴3运动到指定位置
30:
IF iAxis[3].MoveAbs(TRUE,-360,TargetVelFast)  THEN
	iAxis[3].MoveAbs(FALSE,-300,TargetVelFast);
	statecase:=34;
END_IF

// 将轴5运动到指定位置
34:
IF iAxis[5].MoveAbs(TRUE,-360,TargetVelFast)  THEN
	iAxis[5].MoveAbs(FALSE,-300,TargetVelFast);
	statecase:=36;
END_IF

// 将轴5运动回0位
36:
IF iAxis[5].MoveAbs(TRUE,0,TargetVelFast)  THEN
	iAxis[5].MoveAbs(FALSE,0,TargetVelFast);
	statecase:=40;
END_IF

// 将轴3运动回0位
40:
IF iAxis[3].MoveAbs(TRUE,0,TargetVelFast)  THEN
	iAxis[3].MoveAbs(FALSE,0,TargetVelFast);
	statecase:=44;
END_IF

// 将轴1运动回0位
44:
IF iAxis[1].MoveAbs(TRUE,0,TargetVelFast)  THEN
	iAxis[1].MoveAbs(FALSE,0,TargetVelFast);
	statecase:=62;
END_IF


// 将轴3和轴1齿轮耦合，轴1运动到指定位置 
62:
iAxis[3].GearIn(TRUE,iAxis[1],1,1);

IF  iAxis[1].MoveAbs(TRUE,720,TargetVelFast)THEN
	iAxis[1].MoveAbs(FALSE,720,TargetVelFast);
	statecase:=63;
END_IF

// 轴1运动回0位，并解耦轴3
63:
iAxis[3].GearIn(FALSE,iAxis[1],1,1);

IF  iAxis[1].MoveAbs(TRUE,0,TargetVelFast)THEN
	iAxis[1].MoveAbs(FALSE,0,TargetVelFast);
	IF iAxis[3].GearOut(TRUE) THEN
		iAxis[3].GearOut(FALSE);
		statecase:=64;
	END_IF
END_IF

// 将轴3和轴5齿轮耦合，轴5运动到指定位置 
64:
iAxis[3].GearIn(TRUE,iAxis[5],1,1);

IF  iAxis[5].MoveAbs(TRUE,-720,TargetVelFast)THEN
	iAxis[5].MoveAbs(FALSE,-720,TargetVelFast);
	statecase:=65;
END_IF

// 轴5运动回0位，并解耦轴3
65:

iAxis[3].GearIn(FALSE,iAxis[5],1,1);

IF  iAxis[5].MoveAbs(TRUE,0,TargetVelFast)THEN
	iAxis[5].MoveAbs(FALSE,0,TargetVelFast);
	IF iAxis[3].GearOut(TRUE) THEN
		iAxis[3].GearOut(FALSE);
		statecase:=68;
	END_IF
END_IF

// 如果轴5回0位，将234向轴1进行凸轮耦合
68:
IF ((iAxis[5].Nc_To_Plc.ActPos >= -1) AND (iAxis[5].Nc_To_Plc.ActPos <= 1))THEN
	 bCamSwitch	:= TRUE;
END_IF

 IF  bCamSwitch  THEN
	 IF iAxis[2].CamIn(TRUE,iAxis[1],1,2) THEN 
		IF  iAxis[3].CamIn(TRUE,iAxis[1],2,2) THEN
			IF  iAxis[4].CamIn(TRUE,iAxis[1],3,2) THEN
				bCamSwitch:= FALSE;
				statecase:=70;
			END_IF
		END_IF
	 END_IF
 END_IF
 
// 将轴1和轴5移动到指定位置1，这里不需要将轴5和轴1进行凸轮耦合，因为两根轴运动一模一样 
70:
iAxis[2].CamIn(FALSE,iAxis[1],1,2);
iAxis[3].CamIn(FALSE,iAxis[1],2,2);
iAxis[4].CamIn(FALSE,iAxis[1],3,2);

 IF iAxis[1].MoveAbs(TRUE,1440,TargetVelSlow) AND iAxis[5].MoveAbs(TRUE,1440,TargetVelSlow) THEN
	iAxis[1].MoveAbs(FALSE,1440,TargetVelSlow);
	iAxis[5].MoveAbs(FALSE,1440,TargetVelSlow);
	statecase:=72;
 END_IF

// 将轴1和轴5移动到指定位置2
72:
 IF iAxis[1].MoveAbs(TRUE,5040,TargetVelFast) AND iAxis[5].MoveAbs(TRUE,5040,TargetVelFast) THEN
	iAxis[1].MoveAbs(FALSE,5040,TargetVelFast);
	iAxis[5].MoveAbs(FALSE,5040,TargetVelFast);
	statecase:=74;
 END_IF
 
// 将轴1和轴5移动回指定位置 1
74:
 IF iAxis[1].MoveAbs(TRUE,1440,TargetVelFast) AND iAxis[5].MoveAbs(TRUE,1440,TargetVelFast) THEN
	iAxis[1].MoveAbs(FALSE,1440,TargetVelFast);
	iAxis[5].MoveAbs(FALSE,1440,TargetVelFast);
	statecase:=80;
 END_IF

80:
// 将轴1和轴5移动回0位
IF iAxis[1].MoveAbs(TRUE,0,TargetVelSlow) AND iAxis[5].MoveAbs(TRUE,0,TargetVelSlow) THEN
	iAxis[1].MoveAbs(FALSE,0,TargetVelSlow);
	iAxis[5].MoveAbs(FALSE,0,TargetVelSlow);
	statecase:=82; 
END_IF

// 如果轴5回0位了，解耦所有轴
82:
IF ((iAxis[5].Nc_To_Plc.ActPos >= -1) AND (iAxis[5].Nc_To_Plc.ActPos <= 1))THEN
	 bCamSwitch	:= TRUE;
END_IF
 
 IF  bCamSwitch  THEN
	IF iAxis[2].CamOut(TRUE)THEN
		IF iAxis[3].CamOut(TRUE) THEN
			IF iAxis[4].CamOut(TRUE) THEN
				 bCamSwitch	:= FALSE;
				statecase:=90; 
			END_IF
		END_IF
	END_IF	
 END_IF
 
90:
iAxis[2].CamOut(FALSE);
iAxis[3].CamOut(FALSE);
iAxis[4].CamOut(FALSE);
statecase:=500; 

// 停止所有轴，并进入下一个周期 
 500: 
 	IF iAxis[2].Halt(TRUE) AND iAxis[3].Halt(TRUE) AND iAxis[4].Halt(TRUE) THEN
		iAxis[2].Halt(FALSE);
		iAxis[3].Halt(FALSE);
		iAxis[4].Halt(FALSE);
		statecase:=10; 
	END_IF


// 单独回原
840:

IF AxisesHome() THEN
	statecase:=10;
END_IF

// 单独停止运动
1000:
IF iAxis[1].Stop(TRUE) AND iAxis[2].Stop(TRUE) AND iAxis[3].Stop(TRUE) AND iAxis[4].Stop(TRUE) AND iAxis[5].Stop(TRUE) THEN
	iAxis[1].Stop(FALSE);
	iAxis[2].Stop(FALSE);
	iAxis[3].Stop(FALSE);
	iAxis[4].Stop(FALSE);
	iAxis[5].Stop(FALSE);	
END_IF

// 单独复位轴报错	
1010:
IF iAxis[1].Reset(TRUE) AND iAxis[2].Reset(TRUE) AND iAxis[3].Reset(TRUE) AND iAxis[4].Reset(TRUE) AND iAxis[5].Reset(TRUE) THEN
	iAxis[1].Reset(FALSE);
	iAxis[2].Reset(FALSE);
	iAxis[3].Reset(FALSE);
	iAxis[4].Reset(FALSE);
	iAxis[5].Reset(FALSE);	
END_IF

END_CASE


// 停止
IF bStop THEN
	statecase:=1000;
	bStop	:= FALSE;
END_IF

// 复位
IF bReset THEN
	statecase:=1010;
	bReset	:= FALSE;
END_IF

// 启动
IF bStart THEN
	statecase:=0;
	bStart	:= FALSE;
END_IF

// 监控无反应
movingMonitor(in:=iAxis[1].AxesStatus.NotMoving AND (statecase=20) ,PT:=T#5S);
IF movingMonitor.Q  THEN
	iAxis[1].MoveAbs(FALSE,0,TargetVelFast);
	iAxis[2].MoveAbs(FALSE,0,TargetVelFast);
	iAxis[3].MoveAbs(FALSE,0,TargetVelFast);
	iAxis[4].MoveAbs(FALSE,0,TargetVelFast);
	iAxis[5].MoveAbs(FALSE,0,TargetVelFast);
	statecase:=800;
END_IF

// 监控报错
IF Error THEN
	delayton(IN:=TRUE,PT:=T#3S);
	IF delayton.Q THEN
		delayton(IN:=FALSE,PT:=T#3S);
		statecase:=800;
	END_IF
END_IF
END_METHOD

// 运动模式3
METHOD PROTECTED MotionPattern3
VAR_INPUT
END_VAR
;
END_METHOD

PROPERTY P_Reset : BOOL
GET
P_Reset	:= bReset;
END_GET
SET
bReset	:= P_Reset;
END_SET
END_PROPERTY

// 如果为TRUE，启动运行
PROPERTY P_Start : BOOL
GET
P_Start	:= bStart;
END_GET
SET
bStart	:= P_Start;
END_SET
END_PROPERTY

// 如果为TRUE，则停止运动
PROPERTY P_Stop : BOOL
GET
P_Stop	:= bStop;
END_GET
SET
bStop	:= P_Stop;
END_SET
END_PROPERTY

// 运动模式
PROPERTY ShowPattern : INT
GET
ShowPattern	:= _ShowPattern;
END_GET
SET
_ShowPattern	:= ShowPattern;
END_SET
END_PROPERTY

END_FUNCTION_BLOCK

// ---- GlobalTextList.TcGTLO
TEXTLIST GlobalTextList
  634 = '停止'
  856 = '启动'
  255 = '复位'
END_TEXTLIST

// ---- Visus/Visualization.TcVIS
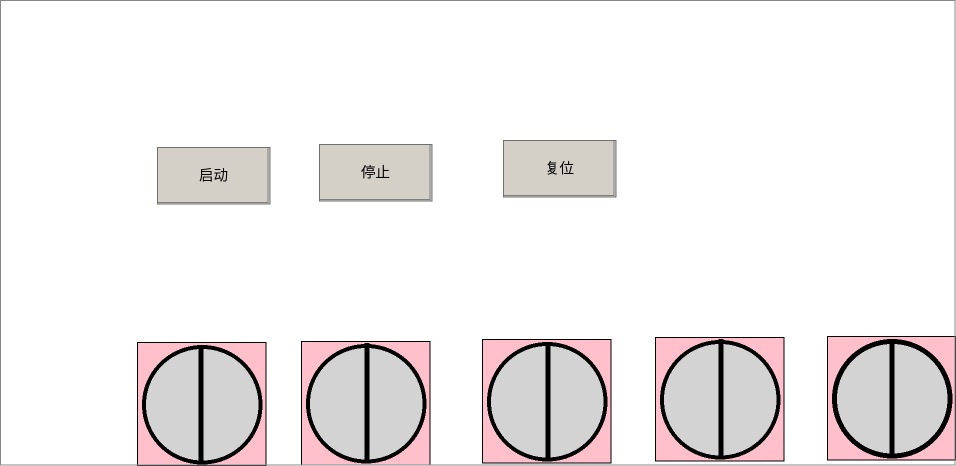
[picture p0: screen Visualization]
VISUALIZATION Visualization  // 956x466
    Textfield (137,342 129x124), invisible if: MAIN.fbVisus.ArrAxisNotMoving[1]
    Ellipse (142,345 120x119)
    Textfield (301,341 129x124), invisible if: MAIN.fbVisus.ArrAxisNotMoving[2]
    Ellipse (306,344 120x119)
    Textfield (482,339 129x124), invisible if: MAIN.fbVisus.ArrAxisNotMoving[3]
    Ellipse (487,342 120x119)
    Textfield (655,337 129x124), invisible if: MAIN.fbVisus.ArrAxisNotMoving[4]
    Ellipse (660,340 120x119)
    Textfield (827,336 129x124), invisible if: MAIN.fbVisus.ArrAxisNotMoving[5]
    Ellipse (832,339 120x119)
    Polyline (201,464) (201,346)
        p2858320360: MAIN.fbVisus.ArrAxisPosition[1]
    Polyline (367,461) (367,343)
        p2858320360: MAIN.fbVisus.ArrAxisPosition[2]
    Polyline (548,461) (548,343)
        p2858320360: MAIN.fbVisus.ArrAxisPosition[3]
    Polyline (721,457) (721,339)
        p2858320360: MAIN.fbVisus.ArrAxisPosition[4]
    Polyline (892,458) (892,340)
        p2858320360: MAIN.fbVisus.ArrAxisPosition[5]
    Button (157,147 113x57), "启动"
        toggle MAIN.bStart
    Button (319,144 113x57), "停止"
        toggle MAIN.bStop
    Button (503,140 113x57), "复位"
        toggle MAIN.bReset
END_VISUALIZATION
